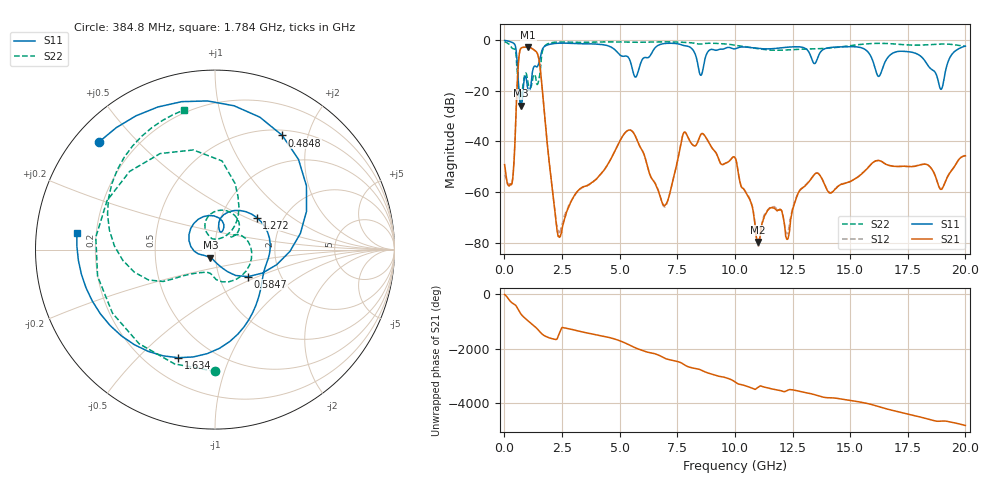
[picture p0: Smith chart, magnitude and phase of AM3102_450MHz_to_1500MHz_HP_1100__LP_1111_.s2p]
!Agilent Technologies,E8364B,MY43040894,A.07.50.67
!Agilent E8364B: A.07.50.67
!Date: Thursday, January 11, 2018 06:36:21
!Correction: S11(Full 2 Port(1,2))
!S21(Full 2 Port(1,2))
!S12(Full 2 Port(1,2))
!S22(Full 2 Port(1,2))
!S2P File: Measurements: S11, S21, S12, S22:
# Hz S  dB  R 50
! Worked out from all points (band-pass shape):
!   1601 points, 10 MHz to 20 GHz, reference 50 ohm
!   highest |S21| = -2.74 dB at 1.034 GHz (marker M1); lowest = -79.8 dB at 10.99 GHz (marker M2)
!   |S21| within 3 dB of the highest: 643.6 MHz to 1.45 GHz (806.7 MHz wide, 77.1 % of centre)
!   lowest |S11| = -25.9 dB at 722.1 MHz (marker M3), VSWR 1.11, Z = 47.4 - j4.2 ohm
!   |S11| at or under -10 dB: 567.5 MHz to 1.457 GHz (889.2 MHz wide, 87.9 % of centre); 16.05 GHz to 16.45 GHz (400 MHz wide, 2.46 % of centre); 18.38 GHz to 19.2 GHz (819 MHz wide, 4.36 % of centre)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
!   |S22| runs from -24.6 to -0.5 dB; largest |S21 - S12| = 0.0017
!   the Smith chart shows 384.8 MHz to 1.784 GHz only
!   S11 on the Smith chart (normalised r, x): 384.8 MHz: 0.07, +0.39; 484.8 MHz: 0.57, +1.60; 584.7 MHz: 1.37, -0.44; 1.272 GHz: 1.47, +0.58; 1.634 GHz: 0.33, -0.66; 1.784 GHz: 0.13, +0.06
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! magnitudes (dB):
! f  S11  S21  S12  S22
! 10 MHz  -0.1  -49.2  -53.1  -0.5
! 384.8 MHz  -1.1  -52.4  -52.5  -3.4
! 484.8 MHz  -2.6  -34.2  -34.2  -4.2
! 584.7 MHz  -12.5  -12.3  -12.3  -15.3
! 722.1 MHz  -25.9  -3.1  -3.2  -24.1
! 1.034 GHz  -19.5  -2.7  -2.7  -17.3
! 1.272 GHz  -10.6  -3.7  -3.7  -13.8
! 1.634 GHz  -3.9  -18.4  -18.4  -5.0
! 1.784 GHz  -2.2  -33.8  -33.8  -2.0
! 2.359 GHz  -1.2  -77.4  -75.6  -0.7
! 3.346 GHz  -1.4  -58.3  -58.4  -0.8
! 5.432 GHz  -7.6  -35.5  -35.5  -0.8
! 6.682 GHz  -2.0  -59.6  -59.5  -0.7
! 7.044 GHz  -1.2  -64.3  -64.7  -0.7
! 7.819 GHz  -2.2  -36.3  -36.3  -0.9
! 10.01 GHz  -3.4  -46.4  -46.4  -2.0
! 10.99 GHz  -3.2  -79.8  -80.9  -3.3
! 12.29 GHz  -2.8  -78.6  -76.3  -3.8
! 13.34 GHz  -7.6  -54.3  -54.4  -3.4
! 16.68 GHz  -6.4  -49.5  -49.4  -1.3
! 18.94 GHz  -19.4  -58.9  -58.7  -1.5
! 20 GHz  -2.3  -45.7  -45.5  -2.4
